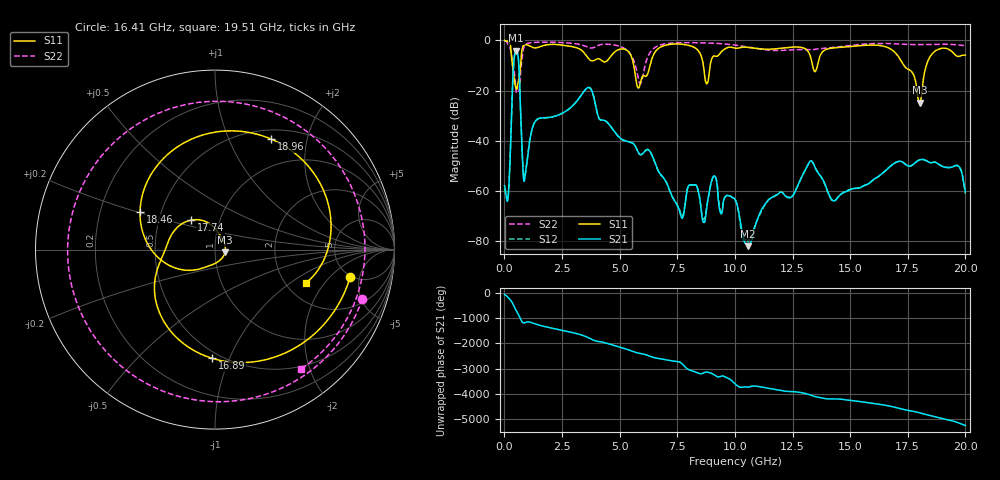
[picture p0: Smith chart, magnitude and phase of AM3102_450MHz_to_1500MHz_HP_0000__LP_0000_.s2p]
!Agilent Technologies,E8364B,MY43040894,A.07.50.67
!Agilent E8364B: A.07.50.67
!Date: Thursday, January 11, 2018 05:13:45
!Correction: S11(Full 2 Port(1,2))
!S21(Full 2 Port(1,2))
!S12(Full 2 Port(1,2))
!S22(Full 2 Port(1,2))
!S2P File: Measurements: S11, S21, S12, S22:
# Hz S  dB  R 50
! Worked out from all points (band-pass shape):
!   1601 points, 10 MHz to 20 GHz, reference 50 ohm
!   highest |S21| = -4.13 dB at 509.8 MHz (marker M1); lowest = -81.9 dB at 10.55 GHz (marker M2)
!   |S21| within 3 dB of the highest: 426.2 MHz to 604.8 MHz (178.6 MHz wide, 34.6 % of centre)
!   lowest |S11| = -24.8 dB at 18.01 GHz (marker M3), VSWR 1.12, Z = 55.9 - j1.6 ohm
!   |S11| at or under -10 dB: 346.4 MHz to 702.5 MHz (356.1 MHz wide, 67.9 % of centre); 5.612 GHz to 6.321 GHz (708.8 MHz wide, 11.9 % of centre); 17.33 GHz to 18.3 GHz (972.4 MHz wide, 5.46 % of centre)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
!   |S22| runs from -20.7 to -0.3 dB; largest |S21 - S12| = 0.0021
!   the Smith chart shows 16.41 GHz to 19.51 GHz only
!   S11 on the Smith chart (normalised r, x): 16.41 GHz: 4.89, -3.62; 16.89 GHz: 0.45, -0.86; 17.74 GHz: 0.73, +0.25; 18.46 GHz: 0.38, +0.20; 18.96 GHz: 0.61, +1.45; 19.51 GHz: 2.53, -1.34
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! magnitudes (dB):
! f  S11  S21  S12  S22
! 10 MHz  -0.1  -57.9  -59.1  -0.3
! 172.4 MHz  -0.6  -61.4  -61.7  -2.0
! 509.8 MHz  -18.7  -4.1  -4.1  -20.2
! 884.6 MHz  -1.8  -54.8  -54.5  -2.0
! 1.359 GHz  -3.0  -32.0  -32.0  -0.8
! 3.346 GHz  -4.0  -21.7  -21.7  -1.8
! 5.82 GHz  -19.0  -44.8  -44.8  -15.7
! 6.682 GHz  -3.3  -52.1  -52.1  -2.1
! 7.694 GHz  -1.6  -70.7  -70.1  -1.0
! 10.01 GHz  -3.1  -63.5  -63.3  -1.9
! 10.55 GHz  -2.8  -81.9  -79.7  -2.7
! 13.34 GHz  -8.7  -48.1  -48.2  -3.8
! 14.27 GHz  -3.1  -63.9  -63.9  -2.8
! 16.41 GHz  -2.3  -52.8  -52.8  -1.3
! 16.68 GHz  -3.1  -50.7  -50.7  -1.3
! 16.89 GHz  -4.4  -49.1  -49.1  -1.4
! 17.74 GHz  -13.5  -49.4  -49.4  -1.7
! 18.01 GHz  -24.8  -47.6  -47.6  -1.7
! 18.46 GHz  -6.6  -48.7  -48.6  -1.7
! 18.96 GHz  -3.2  -50.0  -50.0  -1.6
! 19.51 GHz  -5.4  -50.0  -50.0  -1.7
! 20 GHz  -5.9  -60.1  -61.1  -2.2
